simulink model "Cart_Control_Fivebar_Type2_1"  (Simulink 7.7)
settings: Solver=FixedStepDiscrete  SolverMode=SingleTasking  StartTime=0  StopTime=6  FixedStep=dt  RelTol=1e-3  SampleTimeConstraint=Specified
InitFcn:
  | % Sampling Times %
  | dt0=0.001; dt1=0.01; samples=10;
undefined symbols (not defined in the file or in its folder): DiscIntNeverNeededParam, Volts
libraries: simulink_extras x4, speedgoatlib_IO311 x3, speedgoatlib x2, simulink x2, xpclib x1

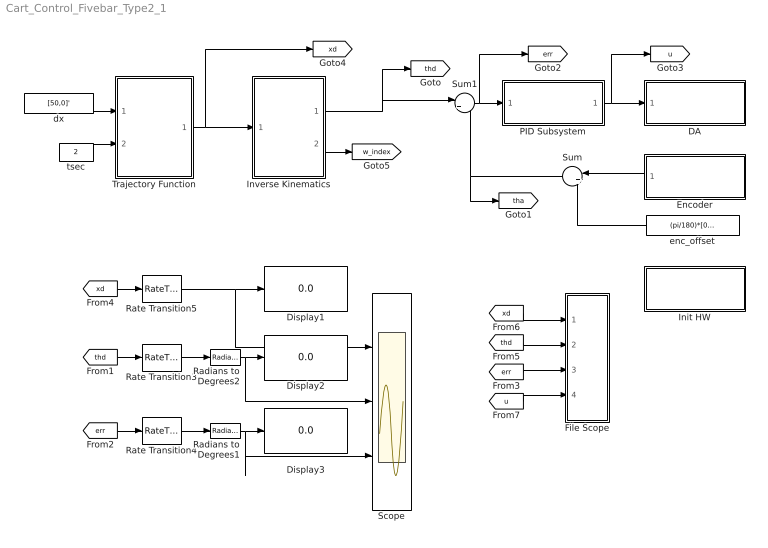
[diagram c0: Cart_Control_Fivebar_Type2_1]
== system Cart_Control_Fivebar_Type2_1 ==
  DA : Subsystem  TreatAsAtomicUnit=on
  Display1 : Display
  Display2 : Display
  Display3 : Display
  Encoder : Subsystem  TreatAsAtomicUnit=on
  File Scope : Subsystem
  Init HW : Subsystem  TreatAsAtomicUnit=on
  Inverse Kinematics : Stateflow chart  TreatAsAtomicUnit=on
  PID Subsystem : Subsystem  TreatAsAtomicUnit=on
  Radians to Degrees1 : simulink_extras/Transformations/Radians to Degrees  SystemSampleTime=-1
  Radians to Degrees2 : simulink_extras/Transformations/Radians to Degrees  SystemSampleTime=-1
  Rate Transition3 : RateTransition  OutPortSampleTime=dt1
  Rate Transition4 : RateTransition  OutPortSampleTime=dt1
  Rate Transition5 : RateTransition  OutPortSampleTime=dt1
  Scope : Scope  NumInputPorts=3
  Sum : Sum  Inputs=|++
  Sum1 : Sum  Inputs=|+-
  Trajectory Function : Stateflow chart  TreatAsAtomicUnit=on
  dx : Constant  Value=[50,0]'  SampleTime=dt0
  enc_offset : Constant  Value=(pi/180)*[0,90]'
  tsec : Constant  Value=2  SampleTime=dt0
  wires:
  Sum1/1 -> [err], PID Subsystem/1(In1)
  PID Subsystem/1(Out1) -> [u], DA/1(In1)
  Encoder/1(Out1) -> Sum/1
  enc_offset/1 -> Sum/2
  Sum/1 -> Sum1/2, [tha]
  [xd] -> File Scope/1(xd)
  [thd] -> File Scope/2(thd)
  [err] -> File Scope/3(err)
  [u] -> File Scope/4(u)
  dx/1 -> Trajectory Function/1(dx)
  tsec/1 -> Trajectory Function/2(tsec)
  Trajectory Function/1(xd) -> [xd], Inverse Kinematics/1(xd)
  Inverse Kinematics/1(thd) -> Sum1/1, [thd]
  [thd] -> Rate Transition3/1
  [err] -> Rate Transition4/1
  [xd] -> Rate Transition5/1
  Rate Transition5/1 -> Display1/1, Scope/1
  Rate Transition3/1 -> Radians to Degrees2/1
  Rate Transition4/1 -> Radians to Degrees1/1
  Radians to Degrees2/1 -> Display2/1, Scope/2
  Radians to Degrees1/1 -> Display3/1, Scope/3
  Inverse Kinematics/2(w_index) -> [w_index]

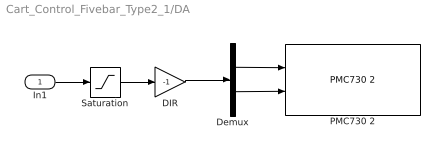
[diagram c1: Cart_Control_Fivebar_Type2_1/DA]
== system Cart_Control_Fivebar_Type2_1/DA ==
  In1 : Inport
  DIR : Gain  Gain=-1
  Demux : Demux  Outputs=2
  PMC730 2 : speedgoatlib/IO101/PMC730 2  id=1  channel=[1,2]  reset=[1,1]  initValue=[0,0]  ts=dt0  pciSlot=-1
  Saturation : Saturate  UpperLimit=10  LowerLimit=-10
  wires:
  In1/1 -> Saturation/1
  Saturation/1 -> DIR/1
  DIR/1 -> Demux/1
  Demux/1 -> PMC730 2/1
  Demux/2 -> PMC730 2/2

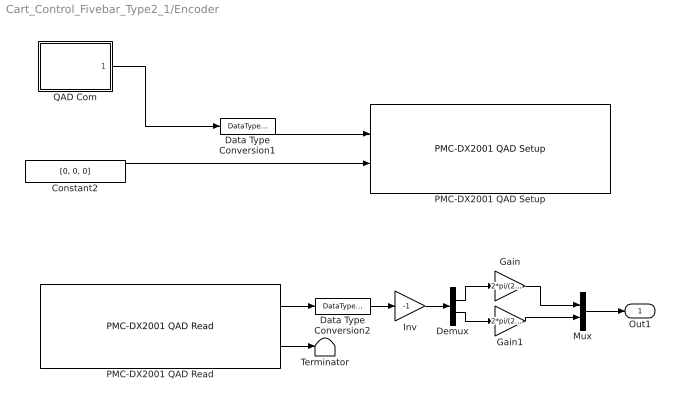
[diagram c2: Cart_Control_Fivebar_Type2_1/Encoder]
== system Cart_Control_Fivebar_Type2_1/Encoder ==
  Constant2 : Constant  Value=[0, 0, 0]  OutDataTypeStr=Inherit: Inherit via back propagation
  Data Type Conversion1 : DataTypeConversion  OutDataTypeStr=uint8
  Data Type Conversion2 : DataTypeConversion  OutDataTypeStr=double
  Demux : Demux  Outputs=2
  Gain : Gain  Gain=2*pi/(23*2000)
  Gain1 : Gain  Gain=2*pi/(23*2000)
  Inv : Gain  Gain=-1
  Mux : Mux  Inputs=2
  PMC-DX2001 QAD Read : speedgoatlib_IO311/PMC-DX2001 QAD Read  id=1  chan=[1, 2]  pciSlot=-1  ts=dt0
  PMC-DX2001 QAD Setup : speedgoatlib_IO311/PMC-DX2001 QAD Setup  id=1  chan=Channel 3 setup  steps1=2000  steps2=2000  steps3=2000  quadrature1=4x  quadrature2=4x  quadrature3=4x  index1=Ignore index input  index2=Ignore index input  index3=Ignore index input  special1=Disabled (cycling counter)  special2=Disabled (cycling counter)  special3=Disabled (cycling counter)  debounce=0  pciSlot=-1  ts=dt0
  QAD Com : Stateflow chart  TreatAsAtomicUnit=on
  Terminator : Terminator
  Out1 : Outport
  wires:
  Constant2/1 -> PMC-DX2001 QAD Setup/2
  PMC-DX2001 QAD Read/2 -> Terminator/1
  PMC-DX2001 QAD Read/1 -> Data Type Conversion2/1
  QAD Com/1(y) -> Data Type Conversion1/1
  Data Type Conversion1/1 -> PMC-DX2001 QAD Setup/1
  Data Type Conversion2/1 -> Inv/1
  Mux/1 -> Out1/1
  Demux/1 -> Gain/1
  Gain/1 -> Mux/1
  Demux/2 -> Gain1/1
  Gain1/1 -> Mux/2
  Inv/1 -> Demux/1

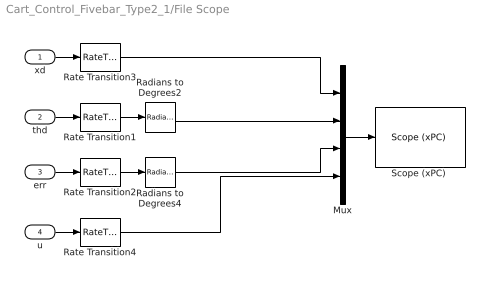
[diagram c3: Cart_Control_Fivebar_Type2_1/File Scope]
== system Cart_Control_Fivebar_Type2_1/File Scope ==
  xd : Inport
  thd : Inport  Port=2
  err : Inport  Port=3
  u : Inport  Port=4
  Mux : Mux
  Radians to Degrees2 : simulink_extras/Transformations/Radians to Degrees  SystemSampleTime=-1
  Radians to Degrees4 : simulink_extras/Transformations/Radians to Degrees  SystemSampleTime=-1
  Rate Transition{1..4} (4 alike) : RateTransition  OutPortSampleTime=dt1
  "Scope (xPC) " : xpclib/Misc./Scope (xPC)   SystemSampleTime=-1  scopeno=1  scopetype=File  autostart=on  viewmode=Graphical redraw  formatstr='%15.6f'  grid=on  ylimits=[0,0]  nosamples=100  noprepostsamples=0  interleave=1  triggermode=FreeRun  triggersignal=1  triggerlevel=0.0  triggerslope=Either  triggerscope=1  triggersample=0  filename=step2.dat  mode=Lazy  writesize=512  autorestart=on  dynamicfilemode=off  maxwritefilesize=512*1024^2
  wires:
  Radians to Degrees2/1 -> Mux/2
  Radians to Degrees4/1 -> Mux/3
  Rate Transition1/1 -> Radians to Degrees2/1
  Rate Transition2/1 -> Radians to Degrees4/1
  thd/1 -> Rate Transition1/1
  err/1 -> Rate Transition2/1
  Rate Transition3/1 -> Mux/1
  xd/1 -> Rate Transition3/1
  u/1 -> Rate Transition4/1
  Mux/1 -> "Scope (xPC) "/1
  Rate Transition4/1 -> Mux/4

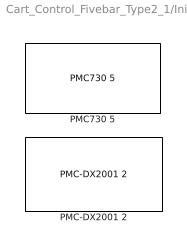
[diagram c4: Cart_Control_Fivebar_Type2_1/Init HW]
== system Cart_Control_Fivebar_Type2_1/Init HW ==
  PMC-DX2001 2 : speedgoatlib_IO311/PMC-DX2001 2  id=1  fpga1=IO311_3PWM_3CAP_3QAD_INT.fpga  fpga2=PWM_Triangle_DX501.fpga  fpga3=PWM_Triangle_DX501.fpga  fpga4=PWM_Triangle_DX501.fpga  fpga5=PWM_Triangle_DX501.fpga  fpga6=PWM_Triangle_DX501.fpga  fpga7=PWM_Triangle_DX501.fpga  fpga8=PWM_Triangle_DX501.fpga  fpga9=PWM_Triangle_DX501.fpga  fpga10=PWM_Triangle_DX501.fpga  group=Module setup  pciSlot=-1  lowerDirection=[ones(1,5), zeros(1, 7), ones(1, 1), ones(1, 3)]  lowerReset=[1]  lowerValue=[0]  upperDirection=[ones(1, 8), zeros(1, 8)]  upperReset=[1]  upperValue=[0]
  PMC730 5 : speedgoatlib/IO101/PMC730 5  id=1  group=Analog output setup  pciSlot=-1  adStartChannel=1  adNumChannel=1  adCoupling=Single-ended  adRange=-10 .. 10 Volts  adAcqMode=Standard  daChannel=[1,2]  daReset=[1,1]  daInitValue=[0,0]  diChannel=[1]  diDebounce=[0]  doChannel=[1]  doReset=[1]  doInitValue=[0]

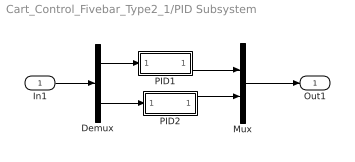
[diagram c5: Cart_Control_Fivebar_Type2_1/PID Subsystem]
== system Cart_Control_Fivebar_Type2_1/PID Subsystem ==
  In1 : Inport
  Demux : Demux  Outputs=2
  Mux : Mux  Inputs=2
  PID1 : Subsystem
  PID2 : Subsystem
  Out1 : Outport
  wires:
  In1/1 -> Demux/1
  Demux/1 -> PID1/1(In1)
  PID1/1(Out1) -> Mux/1
  Demux/2 -> PID2/1(In1)
  PID2/1(Out1) -> Mux/2
  Mux/1 -> Out1/1

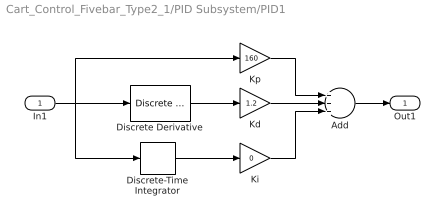
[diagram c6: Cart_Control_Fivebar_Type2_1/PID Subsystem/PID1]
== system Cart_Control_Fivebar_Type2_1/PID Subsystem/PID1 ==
  In1 : Inport
  Add : Sum  Inputs=+++
  Discrete Derivative : simulink/Discrete/Discrete Derivative  SystemSampleTime=-1  gainval=1.0  ICPrevScaledInput=0.0  OutMin=[]  OutMax=[]  OutDataType=fixdt(1, 16)  OutScaling=2^-10  DoSatur=off
  Discrete-Time Integrator : DiscreteIntegrator  SampleTime=dt0  ICPrevOutput=DiscIntNeverNeededParam  ICPrevScaledInput=DiscIntNeverNeededParam
  Kd : Gain  Gain=1.2
  Ki : Gain  Gain=0
  Kp : Gain  Gain=160
  Out1 : Outport
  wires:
  Discrete-Time Integrator/1 -> Ki/1
  Kp/1 -> Add/1
  Kd/1 -> Add/2
  Ki/1 -> Add/3
  Discrete Derivative/1 -> Kd/1
  Add/1 -> Out1/1
  In1/1 -> Kp/1, Discrete Derivative/1, Discrete-Time Integrator/1

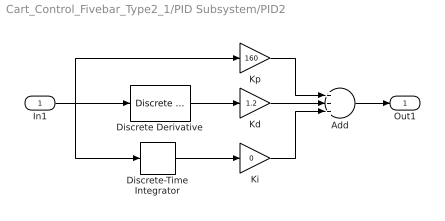
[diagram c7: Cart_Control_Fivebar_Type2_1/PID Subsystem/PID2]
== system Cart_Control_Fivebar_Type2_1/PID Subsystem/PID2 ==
  In1 : Inport
  Add : Sum  Inputs=+++
  Discrete Derivative : simulink/Discrete/Discrete Derivative  SystemSampleTime=-1  gainval=1.0  ICPrevScaledInput=0.0  OutMin=[]  OutMax=[]  OutDataType=fixdt(1, 16)  OutScaling=2^-10  DoSatur=off
  Discrete-Time Integrator : DiscreteIntegrator  SampleTime=dt0  ICPrevOutput=DiscIntNeverNeededParam  ICPrevScaledInput=DiscIntNeverNeededParam
  Kd : Gain  Gain=1.2
  Ki : Gain  Gain=0
  Kp : Gain  Gain=160
  Out1 : Outport
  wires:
  Discrete-Time Integrator/1 -> Ki/1
  Kp/1 -> Add/1
  Kd/1 -> Add/2
  Ki/1 -> Add/3
  Discrete Derivative/1 -> Kd/1
  Add/1 -> Out1/1
  In1/1 -> Kp/1, Discrete Derivative/1, Discrete-Time Integrator/1

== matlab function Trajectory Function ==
function xd = fcn(dx, tsec)

persistent index xd_p

MAX_CH=2;       % Two Actuators %
dt=0.001;       % Step time is 10 msec %

% Initializing Variables %
if isempty(index), index=0; end
if isempty(xd_p), xd_p=zeros(MAX_CH,1); end
xd=zeros(MAX_CH,1);
x0=[100, 128]';

tout=index*dt;
if index<(tsec/dt)
    [c] = coeff_3rd(x0, zeros(MAX_CH,1), x0+dx, zeros(MAX_CH,1), tsec);
    for ch=1:MAX_CH
        xd(ch,1)=c(ch,1)+c(ch,2)*tout+c(ch,3)*tout^2+c(ch,4)*tout^3;    
    end
    xd_p=xd;
else
    xd=xd_p;
end
index=index+1;

function [c] = coeff_3rd(sp, sv, ep, ev, tsec)
MAX_CH=2;
c=zeros(MAX_CH,4);
for ch=1:MAX_CH
    c(ch,1)=sp(ch,1);
    c(ch,2)=sv(ch,1);
    c(ch,3)=(3.0*(ep(ch,1)-sp(ch,1))-(2.0*sv(ch,1)+ev(ch,1))*tsec)/(tsec*tsec);
    c(ch,4)=(-2.0*(ep(ch,1)-sp(ch,1))+(sv(ch,1)+ev(ch,1))*tsec)/(tsec*tsec*tsec);
end

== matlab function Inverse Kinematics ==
function [thd,w_index]  = fcn(xd)

persistent index thd_p
persistent th3_p th4_p

% Initializing Variables %
if isempty(index), index=0; end
if isempty(thd_p), thd_p=(pi/180)*[0,90]'; end
if isempty(th3_p), th3_p=0; end
if isempty(th4_p), th4_p=0; end

% Kinematic Parameters %
L1=200; L2=100; L3=100; L4=100; L5=100; L6=28;

w_index=1;  % In workspace %

% (1) Left Side 2-DOF Arm %
px=xd(1,1); py=xd(2,1);
k1=(px^2+py^2-L2^2-(L3+L6)^2)/(2*L2*(L3+L6));
if abs(k1)<=1
    th3=+acos(k1);  % Note the sign %
else
    w_index=-1;
    th3=th3_p;
end

DEL1=L2^2+(L3+L6)^2+2*L2*(L3+L6)*cos(th3);
cth2=(px*(L2+(L3+L6)*cos(th3))+py*(L3+L6)*sin(th3))/DEL1;
sth2=(-px*(L3+L6)*sin(th3)+py*(L2+(L3+L6)*cos(th3)))/DEL1;
th2=atan2(sth2,cth2);

% (2) Right Side 2-DOF Arm %
cx=px-L6*cos(th2+th3)-L1; cy=py-L6*sin(th2+th3);
k2=(cx^2+cy^2-L5^2-L4^2)/(2*L5*L4);
if abs(k2)<=1
    th4=acos(k2);
else
    w_index=-2;
    th4=th4_p;
end

DEL2=L5^2+L4^2+2*L5*L4*cos(th4);
cth5=(cx*(L5+L4*cos(th4))+cy*L4*sin(th4))/DEL2;
sth5=(-cx*L4*sin(th4)+cy*(L5+L4*cos(th4)))/DEL2;
th5=atan2(sth5,cth5);

% Result %
if w_index==1
    thd=[th2, th5]';
else
    thd=thd_p;
end

% Save the current value %
thd_p=thd;
th3_p=th3; th4_p=th4;

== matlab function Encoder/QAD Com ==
function y = fcn()

persistent index

if isempty(index), index=0; end

if index==0
    y=[1,1,1];      %  Reset %
else
    y = [0,0,0];
end

index=index+1;
